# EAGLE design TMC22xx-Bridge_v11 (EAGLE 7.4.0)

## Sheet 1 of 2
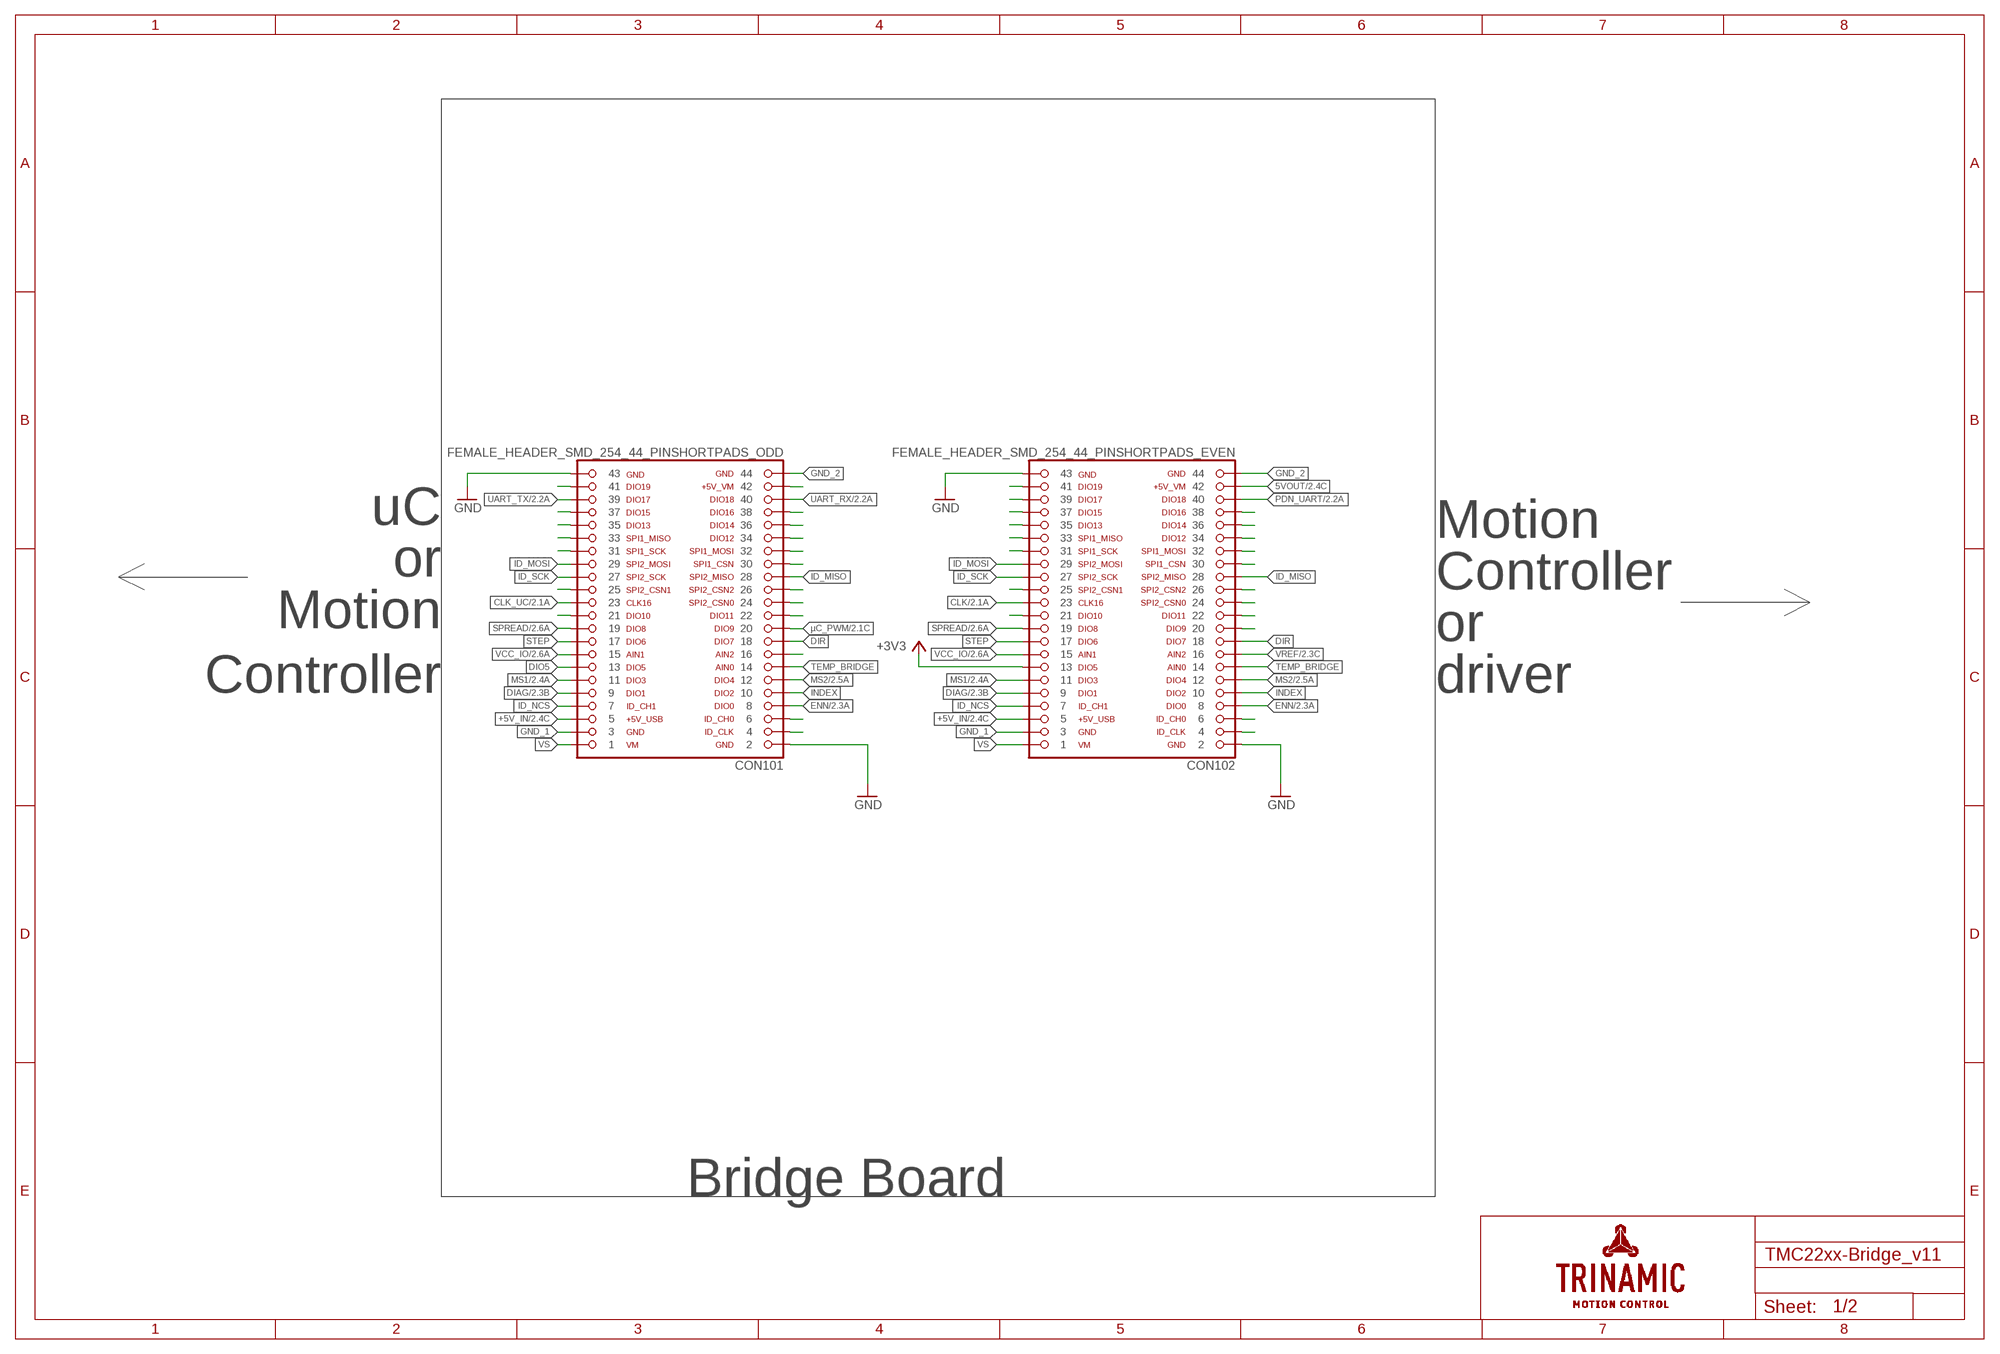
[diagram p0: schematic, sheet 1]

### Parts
CON101  FEMALE_HEADER_SMD_254_44_PINSHORTPADS_ODD  FEMALE_HEADER_SMD_2.54_44_PIN_BRIDGEESELSBRUECKE_ODD  [MALE_HEADER_SMD_254_44_PIN_SHORTPADS_ODD]
CON102  FEMALE_HEADER_SMD_254_44_PINSHORTPADS_EVEN  FEMALE_HEADER_SMD_2.54_44_PIN_BRIDGEESELSBRUECKE_EVEN  [MALE_HEADER_SMD_254_44_PIN_SHORTPADS_EVEN]

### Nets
5VOUT: CON102.1@42 CON102.42 ; also sheet 2
+3V3: CON102.13 ; also sheet 2
+5V_IN: CON101.1@5 CON101.5 CON102.5 ; also sheet 2
CLK: CON102.23 ; also sheet 2
CLK_UC: CON101.1@23 CON101.23 ; also sheet 2
DIAG: CON101.1@9 CON101.9 CON102.9 ; also sheet 2
DIO5: CON101.1@13 CON101.13
DIR: CON101.18 CON102.1@18 CON102.18
ENN: CON101.8 CON102.1@8 CON102.8 ; also sheet 2
GND: CON101.1@43 CON101.2 CON101.43 CON102.1@2 CON102.2 CON102.43 ; also sheet 2
GND_1: CON101.1@3 CON101.3 CON102.3
GND_2: CON101.44 CON102.1@44 CON102.44
ID_MISO: CON101.28 CON102.1@28 CON102.28
ID_MOSI: CON101.1@29 CON101.29 CON102.29
ID_NCS: CON101.1@7 CON101.7 CON102.7
ID_SCK: CON101.1@27 CON101.27 CON102.27
INDEX: CON101.10 CON102.1@10 CON102.10
MS1: CON101.1@11 CON101.11 CON102.11 ; also sheet 2
MS2: CON101.12 CON102.1@12 CON102.12 ; also sheet 2
N$4: CON101.1@41 CON101.41
N$6: CON101.1@37 CON101.37
N$7: CON101.1@35 CON101.35
N$8: CON101.1@33 CON101.33
N$9: CON101.1@31 CON101.31
N$10: CON101.1@25 CON101.25
N$11: CON101.1@21 CON101.21
N$13: CON101.4
N$14: CON101.6
N$15: CON101.22
N$16: CON101.26
N$17: CON101.24
N$18: CON101.30
N$19: CON101.32
N$20: CON101.34
N$21: CON101.36
N$22: CON101.38
N$23: CON101.42
N$24: CON102.41
N$25: CON102.39
N$26: CON102.37
N$27: CON102.35
N$28: CON102.33
N$29: CON102.31
N$30: CON102.25
N$31: CON102.21
N$33: CON102.1@4 CON102.4
N$34: CON102.1@6 CON102.6
N$35: CON102.1@20 CON102.20
N$36: CON102.1@22 CON102.22
N$37: CON102.1@24 CON102.24
N$38: CON102.1@26 CON102.26
N$39: CON102.1@30 CON102.30
N$40: CON102.1@32 CON102.32
N$41: CON102.1@34 CON102.34
N$42: CON102.1@36 CON102.36
N$43: CON102.1@38 CON102.38
PDN_UART: CON102.1@40 CON102.40 ; also sheet 2
SPREAD: CON101.1@19 CON101.19 CON102.19 ; also sheet 2
STEP: CON101.1@17 CON101.17 CON102.17
TEMP_BRIDGE: CON101.14 CON102.1@14 CON102.14
UART_RX: CON101.40 ; also sheet 2
UART_TX: CON101.1@39 CON101.39 ; also sheet 2
VCC_IO: CON101.1@15 CON101.15 CON102.15 ; also sheet 2
VREF: CON102.1@16 CON102.16 ; also sheet 2
VREF_NC: CON101.16
VS: CON101.1 CON101.1@1 CON102.1
µC_PWM: CON101.20 ; also sheet 2

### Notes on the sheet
- uC
- or | Motion
- Motion | Controller
- Controller | or
- driver
- Bridge Board

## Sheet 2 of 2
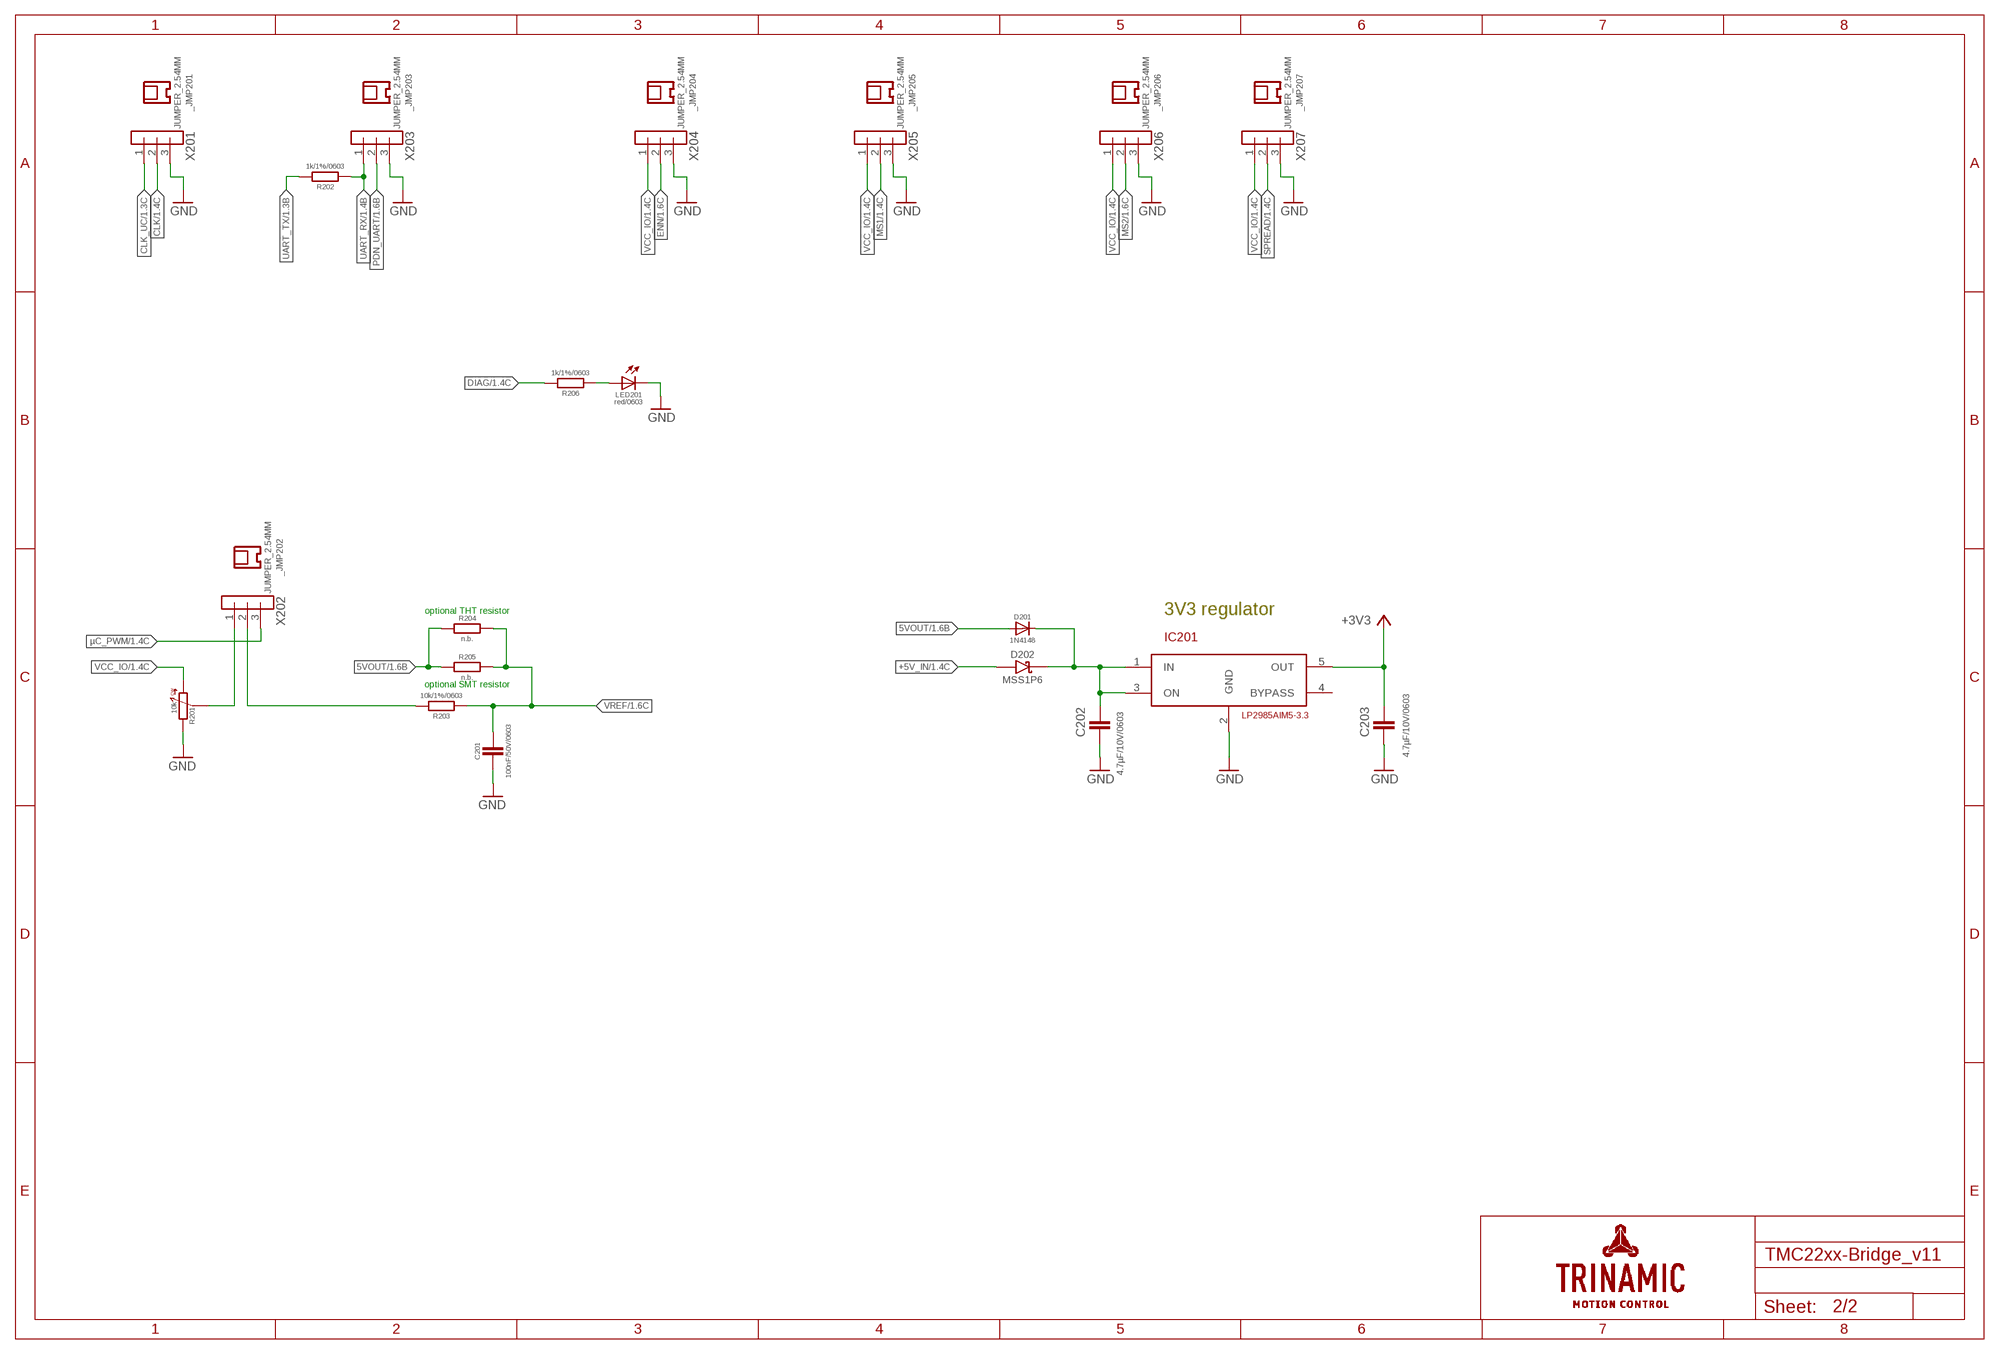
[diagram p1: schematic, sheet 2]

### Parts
_JMP201  JUMPER_2.54MM  [JUMPER_DOKU]
_JMP202  JUMPER_2.54MM  [JUMPER_DOKU]
_JMP203  JUMPER_2.54MM  [JUMPER_DOKU]
_JMP204  JUMPER_2.54MM  [JUMPER_DOKU]
_JMP205  JUMPER_2.54MM  [JUMPER_DOKU]
_JMP206  JUMPER_2.54MM  [JUMPER_DOKU]
_JMP207  JUMPER_2.54MM  [JUMPER_DOKU]
C201  100nF/50V/0603  C0603  [_RC_0603]
C202  4.7µF/10V/0603  C0603  [_RC_0603]
C203  4.7µF/10V/0603  C0603  [_RC_0603]
D201  1N4148  [D0603]
D202  MSS1P6  [MICROSMP]
IC201  LP2985AIM5-3.3  [SOT23-5]
LED201  red/0603  LED0603  [_D_0603]
R201  10k  CT-6EP  [COPAL-CT-6]
R202  1k/1%/0603  R0603  [_RC_0603]
R203  10k/1%/0603  R0603  [_RC_0603]
R204  n.b.  R-EU_0613/5V  [P0613V]
R205  n.b.  R_NOCREAM  [_RC_1206_NOCREAM]
R206  1k/1%/0603  R0603  [_RC_0603]
X201  3PIN_1ROWTHT  [3PIN_1ROM_2,54_THT]
X202  3PIN_1ROWTHT  [3PIN_1ROM_2,54_THT]
X203  3PIN_1ROWTHT  [3PIN_1ROM_2,54_THT]
X204  3PIN_1ROWTHT  [3PIN_1ROM_2,54_THT]
X205  3PIN_1ROWTHT  [3PIN_1ROM_2,54_THT]
X206  3PIN_1ROWTHT  [3PIN_1ROM_2,54_THT]
X207  3PIN_1ROWTHT  [3PIN_1ROM_2,54_THT]

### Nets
5V_TO_REG: C202.P$1 D201.K(C) D202.C IC201.1(IN) IC201.3(ON)
5VOUT: D201.A R204.1 R205.P$1 ; also sheet 1
+3V3: C203.P$1 IC201.5(OUT) ; also sheet 1
+5V_IN: D202.A ; also sheet 1
CLK: X201.2 ; also sheet 1
CLK_UC: X201.1 ; also sheet 1
DIAG: R206.P$2 ; also sheet 1
ENN: X204.2 ; also sheet 1
GND: C201.P$2 C202.P$2 C203.P$2 IC201.2(GND) LED201.C R201.P$1 X201.3 X203.3 X204.3 X205.3 X206.3 X207.3 ; also sheet 1
MS1: X205.2 ; also sheet 1
MS2: X206.2 ; also sheet 1
N$5: LED201.A R206.P$1
PDN_UART: X203.2 ; also sheet 1
SPREAD: X207.2 ; also sheet 1
UART_RX: R202.P$1 X203.1 ; also sheet 1
UART_TX: R202.P$2 ; also sheet 1
VCC_IO: R201.P$3 X204.1 X205.1 X206.1 X207.1 ; also sheet 1
VREF: C201.P$1 R203.P$1 R204.2 R205.P$2 ; also sheet 1
VREF_POT: R201.P$2 X202.1
VREF_POT_JP: R203.P$2 X202.2
µC_PWM: X202.3 ; also sheet 1
Unconnected: IC201.4(BYPASS)

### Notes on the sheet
- optional THT resistor | 3V3 regulator
- optional SMT resistor

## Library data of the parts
_JMP201-_JMP207 = TMC2208-Eval:JUMPER_2.54MM: Jumper 2.54mm, Open top, h6.5mm, black
C201-C203 = TMC2208-Eval:C
CON101 CON102 = TMC2208-Eval:FEMALE_HEADER_SMD_2.54_44_PIN_BRIDGE; SUPPLIER: MPE Garry; SUPPLIER-CODE: 090-3-044-1-F-XT0-0910
D201 = TMC2208-Eval:1N4148: DIODE; OC_DIGIKEY: 641-1001-1-ND; SUPPLIER: DigiKey; SUPPLIER-CODE: 641-1001-1-ND
D202 = TMC2208-Eval:MSS1P6; OC_DIGIKEY: MSS1P6-M3/89AGICT-ND; SUPPLIER: DigiKey; SUPPLIER-CODE: MSS1P6-M3/89AGICT-ND
IC201 = TMC2208-Eval:LP2985AIM5-3.3; OC_DIGIKEY: LP2985AIM5-3.3/NOPBCT-ND; SUPPLIER: DigiKey; SUPPLIER-CODE: LP2985AIM5-3.3/NOPBCT-ND
LED201 = TMC2208-Eval:LED
R201 = TMC2208-Eval:CT-6EP: Copal CT-6EP Potentiometer; OC_DIGIKEY: CT6EP103-ND; SUPPLIER: DigiKey; SUPPLIER-CODE: CT6EP103-ND
R202 R203 R206 = TMC2208-Eval:R
R204 = TMC2208-Eval:R-EU_: RESISTOR, European symbol
R205 = TMC2208-Eval:R_NOCREAM
X201-X207 = TMC2208-Eval:3PIN_1ROW

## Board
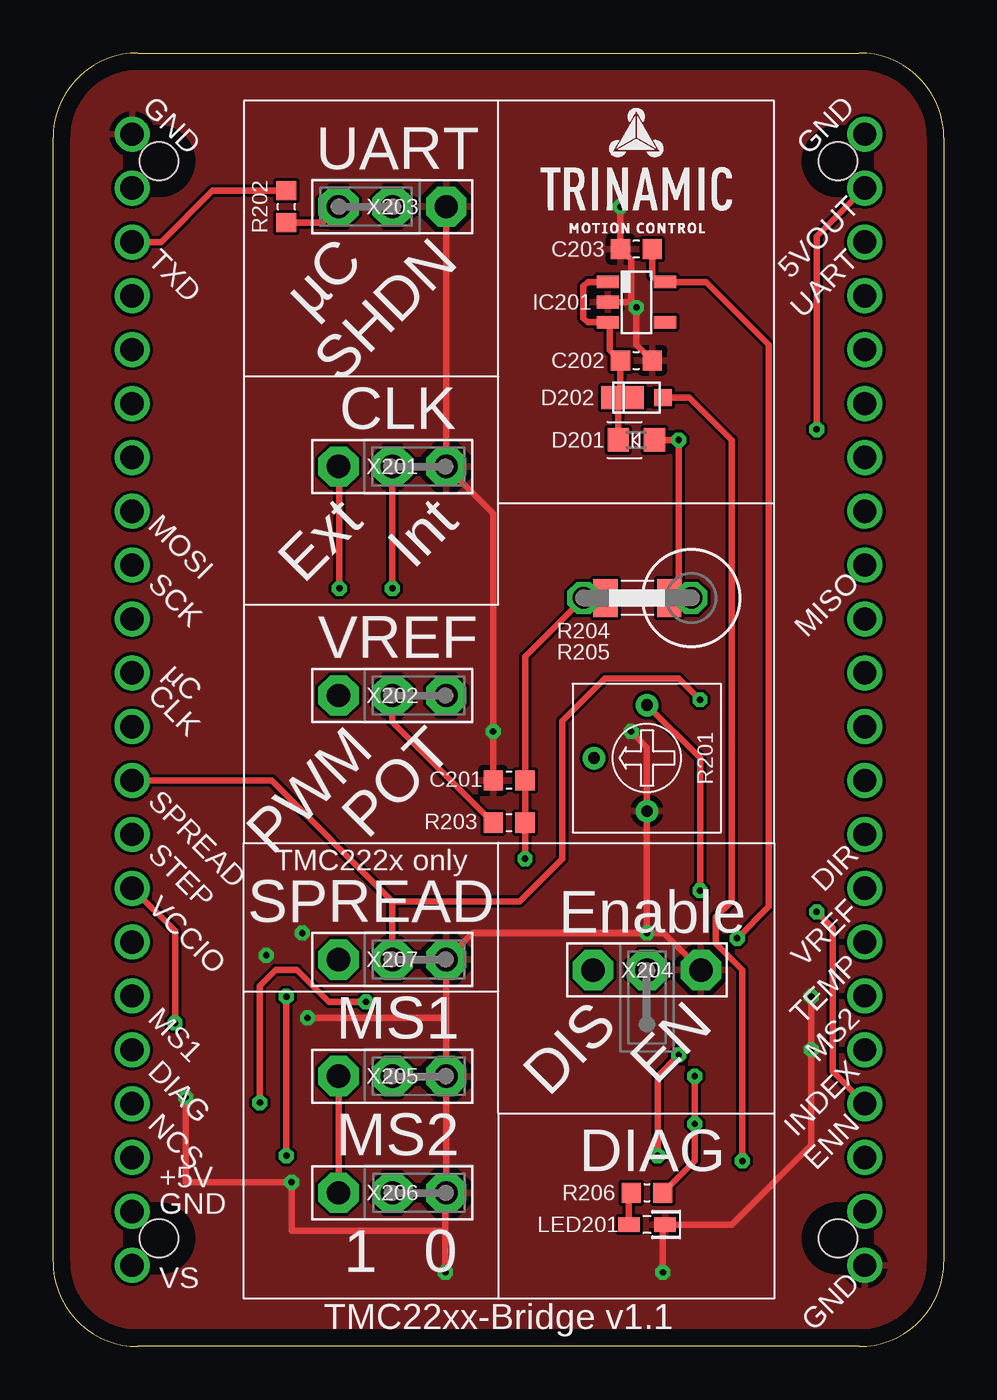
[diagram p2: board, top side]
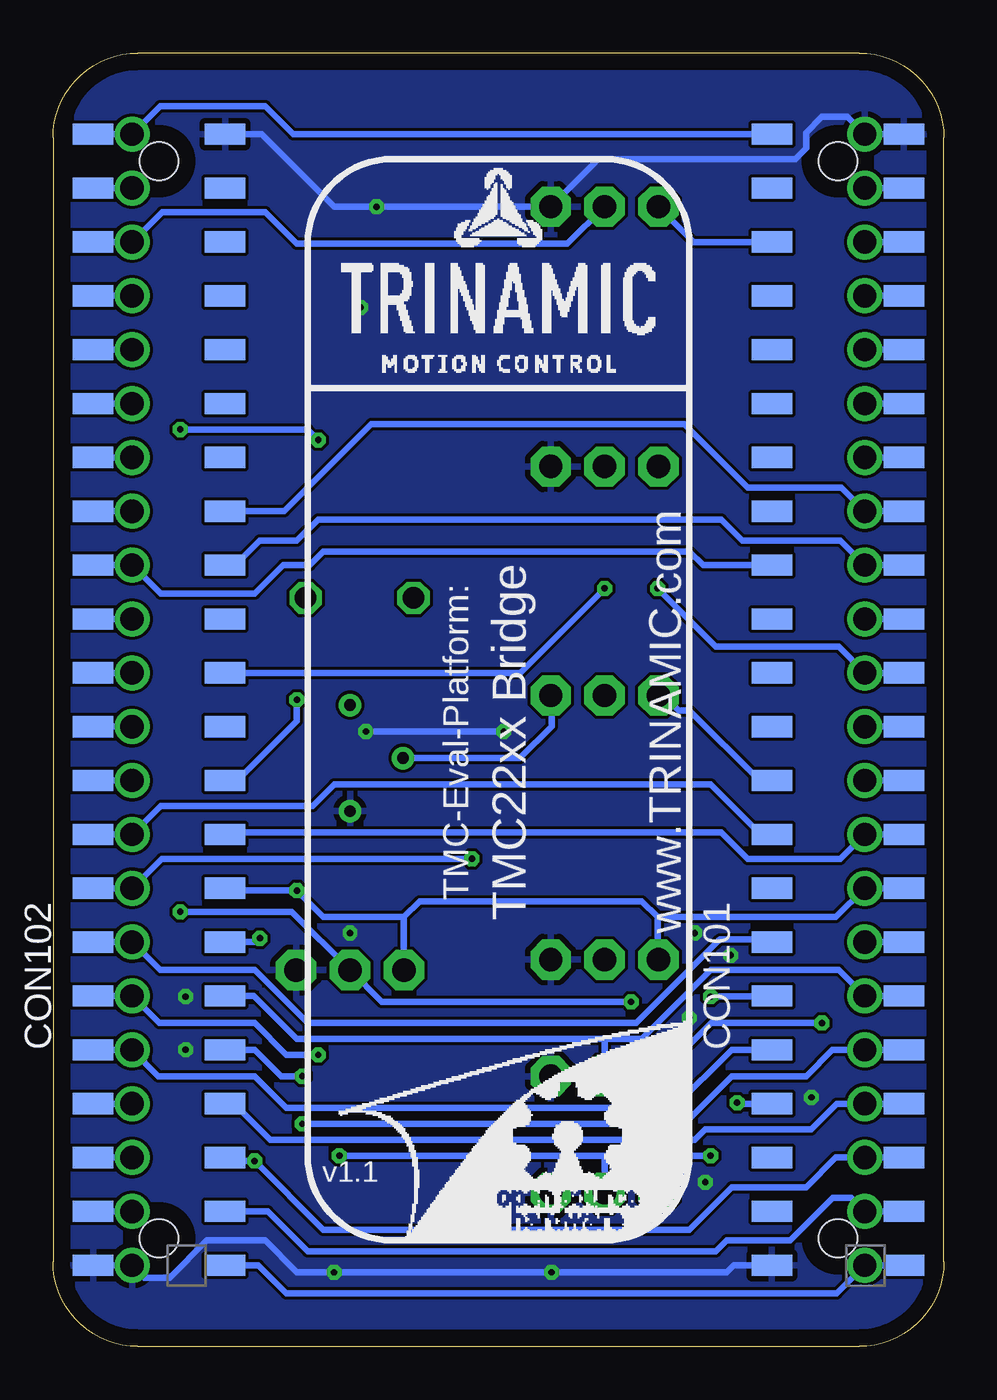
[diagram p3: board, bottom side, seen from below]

Size 42 x 61 mm. Coordinates in mm from the lower left corner, seen from the top.
Outline: 38,0 4,0 arc-90 0,4 0,57 arc-90 4,61 38,61 arc-90 42,57 42,4 arc-90 38,0
Copper layers (1*16): Top 0.018mm / dielectric 0.36mm / Bottom 0.018mm
Design rules "default": minimum track width 0.15mm, minimum drill 0.25mm, track to track 0.15mm, track to pad 0.15mm, pad to pad 0.1mm, via to via 0.15mm, smd to smd 0mil, copper to edge 0.8mm, drill to drill 8mil, minimum pad ring 10mil, minimum via ring 8mil, stop-mask expansion 4mil, vias tented up to drill 0.4mm, thermal gap 10mil

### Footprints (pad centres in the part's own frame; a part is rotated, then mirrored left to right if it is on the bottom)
_RC_0603 = smd 0.9 x 0.95: P$1 -0.75,0; P$2 0.75,0
MALE_HEADER_SMD_254_44_PIN_SHORTPADS_ODD = smd 1 x 1.9: 1 -26.67,-3.11; 2 -26.67,3.11; 3 -24.13,-3.11; 4 -24.13,3.11; 5 -21.59,-3.11; 6 -21.59,3.11; 7 -19.05,-3.11; 8 -19.05,3.11; 9 -16.51,-3.11; 10 -16.51,3.11; 11 -13.97,-3.11; 12 -13.97,3.11; 13 -11.43,-3.11; 14 -11.43,3.11; 15 -8.89,-3.11; 16 -8.89,3.11; 17 -6.35,-3.11; 18 -6.35,3.11; 19 -3.81,-3.11; 20 -3.81,3.11; 21 -1.27,-3.11; 22 -1.27,3.11; 23 1.27,-3.11; 24 1.27,3.11; 25 3.81,-3.11; 26 3.81,3.11; 27 6.35,-3.11; 28 6.35,3.11; 29 8.89,-3.11; 30 8.89,3.11; 31 11.43,-3.11; 32 11.43,3.11; 33 13.97,-3.11; 34 13.97,3.11; 35 16.51,-3.11; 36 16.51,3.11; 37 19.05,-3.11; 38 19.05,3.11; 39 21.59,-3.11; 40 21.59,3.11; 41 24.13,-3.11; 42 24.13,3.11; 43 26.67,-3.11; 44 26.67,3.11 | drill 1.1 pad 1.45: 1@1 -26.67,-1.27; 1@3 -24.13,-1.27; 1@5 -21.59,-1.27; 1@7 -19.05,-1.27; 1@9 -16.51,-1.27; 1@11 -13.97,-1.27; 1@13 -11.43,-1.27; 1@15 -8.89,-1.27; 1@17 -6.35,-1.27; 1@19 -3.81,-1.27; 1@21 -1.27,-1.27; 1@23 1.27,-1.27; 1@25 3.81,-1.27; 1@27 6.35,-1.27; 1@29 8.89,-1.27; 1@31 11.43,-1.27; 1@33 13.97,-1.27; 1@35 16.51,-1.27; 1@37 19.05,-1.27; 1@39 21.59,-1.27; 1@41 24.13,-1.27; 1@43 26.67,-1.27 | hole 1.8: -25.4,0; 25.4,0
MALE_HEADER_SMD_254_44_PIN_SHORTPADS_EVEN = smd 1 x 1.9: 1 -26.67,-3.11; 2 -26.67,3.11; 3 -24.13,-3.11; 4 -24.13,3.11; 5 -21.59,-3.11; 6 -21.59,3.11; 7 -19.05,-3.11; 8 -19.05,3.11; 9 -16.51,-3.11; 10 -16.51,3.11; 11 -13.97,-3.11; 12 -13.97,3.11; 13 -11.43,-3.11; 14 -11.43,3.11; 15 -8.89,-3.11; 16 -8.89,3.11; 17 -6.35,-3.11; 18 -6.35,3.11; 19 -3.81,-3.11; 20 -3.81,3.11; 21 -1.27,-3.11; 22 -1.27,3.11; 23 1.27,-3.11; 24 1.27,3.11; 25 3.81,-3.11; 26 3.81,3.11; 27 6.35,-3.11; 28 6.35,3.11; 29 8.89,-3.11; 30 8.89,3.11; 31 11.43,-3.11; 32 11.43,3.11; 33 13.97,-3.11; 34 13.97,3.11; 35 16.51,-3.11; 36 16.51,3.11; 37 19.05,-3.11; 38 19.05,3.11; 39 21.59,-3.11; 40 21.59,3.11; 41 24.13,-3.11; 42 24.13,3.11; 43 26.67,-3.11; 44 26.67,3.11 | drill 1.1 pad 1.45: 1@2 -26.67,1.27; 1@4 -24.13,1.27; 1@6 -21.59,1.27; 1@8 -19.05,1.27; 1@10 -16.51,1.27; 1@12 -13.97,1.27; 1@14 -11.43,1.27; 1@16 -8.89,1.27; 1@18 -6.35,1.27; 1@20 -3.81,1.27; 1@22 -1.27,1.27; 1@24 1.27,1.27; 1@26 3.81,1.27; 1@28 6.35,1.27; 1@30 8.89,1.27; 1@32 11.43,1.27; 1@34 13.97,1.27; 1@36 16.51,1.27; 1@38 19.05,1.27; 1@40 21.59,1.27; 1@42 24.13,1.27; 1@44 26.67,1.27 | hole 1.8: -25.4,0; 25.4,0
D0603 = smd 1 x 1.1: A -0.85,0; K 0.85,0
MICROSMP = smd 0.813 x 0.813: A 1.257,0 | smd 2.007 x 1.092: C -0.66,0
SOT23-5 = smd 0.6 x 1.05: 1 -0.95,-1.35; 2 0,-1.35; 3 0.95,-1.35; 4 0.95,1.35; 5 -0.95,1.35
_D_0603 = smd 1 x 0.7: A 0.85,0; C -0.85,0
COPAL-CT-6 = drill 0.55: P$1 -2.5,0; P$2 0,2.5; P$3 2.5,0
P0613V = drill 1.016 octagon: 1 -2.54,0; 2 2.54,0
_RC_1206_NOCREAM = smd 1.15 x 1.8: P$1 -1.5,0; P$2 1.5,0
3PIN_1ROM_2,54_THT = drill 1.1 pad 1.9 octagon: 1 -2.54,0; 2 0,0; 3 2.54,0

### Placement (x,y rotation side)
_JMP201  17.23,18.25 0 top
_JMP202  28,16.46 90 top
_JMP203  17.24,12.75 0 top
_JMP204  17.25,7.25 0 top
_JMP205  17.23,30.7 0 top
_JMP206  17.22,41.5 0 top
_JMP207  14.75,53.75 0 top
C201  21.5,26.7 180 top
C202  27.5,46.5 0 top
C203  27.5,51.75 180 top
CON101  5,30.5 90 bottom
CON102  37,30.5 90 bottom
D201  27.5,42.75 180 top
D202  27.5,44.75 0 top
IC201  27.5,49.25 270 top
LED201  28,5.75 180 top
R201  28,27.75 90 top
R202  11,53.75 90 top
R203  21.5,24.7 180 top
R204  27.55,35.3 180 top
R205  27.55,35.3 180 top
R206  28,7.25 0 top
U$3  [TRINAMIC_LOGO]  23,52.5 0 top
U$4  [TMC_EVAL_BACK_BRIDGE]  30,5 0 bottom
X201  16,41.5 0 top
X202  16,30.7 180 top
X203  16,53.75 0 top
X204  28,17.75 0 top
X205  16,12.75 0 top
X206  16,7.25 0 top
X207  16,18.25 0 top

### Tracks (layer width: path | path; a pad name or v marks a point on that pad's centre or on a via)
5V_TO_REG
  Top 0.3: IC201.1 25.2,50.2 25,50 25,48.5 25.2,48.3 IC201.3 26.25,48.2 26.25,47 C202.P$1 26.75,44.84 D202.C 26.65,44.56 D201.K
5VOUT  (via drill 0.3)
  Top 0.3: R204.1 R205.P$1 29.5,35.75 v29.5,42.75 D201.A | CON102.1@42 36,52.36 v36,43.25
  Bottom 0.3: CON102.42 CON102.1@42 | v36,43.25 30,43.25 v29.5,42.75
+3V3  (via drill 0.3)
  Top 0.3: C203.P$1 28.25,50.5 28.55,50.2 IC201.5 30.8,50.2 33.75,47.25 33.75,20.75 v32.25,19.25
  Bottom 0.3: CON102.13 32.43,19.07 v32.25,19.25
+5V_IN  (via drill 0.3)
  Top 0.3: v32.5,8.75 32.5,17.75 31.25,19 31.25,20.25 32,21 32,42.75 30,44.75 D202.A
  Bottom 0.3: CON101.5 CON101.1@5 5.09,8.91 6.5,7.5 10,7.5 12,5.5 29.25,5.5 v32.5,8.75 33.73,8.75 CON102.5
CLK  (via drill 0.3)
  Top 0.3: v16,35.75 X201.2
  Bottom 0.3: 33.87,31.75 CON102.23 19.98,31.77 v16,35.75
CLK_UC  (via drill 0.3)
  Top 0.3: X201.1 13.5,41.46 v13.5,35.75
  Bottom 0.3: CON101.23 CON101.1@23 4.96,33 10.75,33 v13.5,35.75
DIAG  (via drill 0.3)
  Top 0.3: R206.P$2 30.25,8.75 v30.25,10.5 v30.25,12.75
  Bottom 0.3: CON101.9 CON101.1@9 5.26,13.99 6.5,12.75 10,12.75 12.25,10.5 v30.25,10.5 | CON102.9 32.49,13.99 31.25,12.75 v30.25,12.75
DIO5
  Bottom 0.3: CON101.13 CON101.1@13
DIR
  Bottom 0.3: CON102.18 CON102.1@18 36.92,25.5 29.75,25.5 28.75,26.5 11,26.5 8.5,24 8.26,24 CON101.18
ENN  (via drill 0.3)
  Top 0.3: v36,20.5 36.75,19.75 36.75,12.97 CON102.1@8 | v14.75,16.25 13,16.25 11.5,17.75 10.5,17.75 9.75,17 v9.75,11.5
  Bottom 0.3: CON102.8 CON102.1@8 | v36,20.5 30.75,20.5 X204.2 26.5,16.25 v14.75,16.25 | v9.75,11.5 9.7,11.45 CON101.8
GND  (via drill 0.3)
  Top 0.3: 27.25,49.25 27.25,51.25 C203.P$2 v26.75,53.75 | 27.25,49.25 IC201.2 | C202.P$2 27.5,47.25 v27.5,49 27.25,49.25 | C201.P$2 v20.75,29 20.75,39.29 X201.3 X203.3 | v27.25,29 28,28.25 R201.P$1 v28,19.5 | v28.75,3.5 28.75,5.65 LED201.C 32,5.75 35.75,9.5 v35.75,14 v35.75,16.5 | 18.5,5.45 18.5,7.21 X206.3 X205.3 18.54,15.5 | 18.5,5.45 v18.5,3.5 | v28,19.5 19.79,19.5 X207.3 18.54,15.5 | X204.3 28.79,19.5 v28,19.5 | 18.54,15.5 v12,15.5 | 18.5,5.45 11.25,5.45 v11.25,7.75 6.25,7.75 v6.25,11.75
  Bottom 0.3: CON101.43 CON101.1@43 4.56,58 5.75,58 6.5,57.25 6.5,56.5 7,56 16.29,56 X203.3 v26.75,53.75 28.75,53.75 32.17,57.17 CON102.43 | v27.25,29 v20.75,29 | CON102.2 CON102.1@2 37.69,3.25 36.5,3.25 34.75,5 32,5 30.5,3.5 v28.75,3.5 v18.5,3.5 10.25,3.5 9.92,3.83 CON101.2
  other vias: 11.75,19.5 10.05,18.45
  pour Bottom: 42,61 0,61 0,0 42,0
  pour Top: 42,61 0,61 0,0 42,0
GND_1
  Bottom 0.3: CON101.3 CON101.1@3 4.36,7 5.25,7 7.25,5 10.25,5 10.75,4.5 30,4.5 31.87,6.37 CON102.3
GND_2
  Bottom 0.3: CON102.44 CON102.1@44 36.94,58.5 32,58.5 30.67,57.17 CON101.44
ID_MISO
  Bottom 0.3: CON102.28 CON102.1@28 36.92,35.5 32.5,35.5 31.15,36.85 29.9,36.85 29.25,37.5 12,37.5 11.35,36.85 CON101.28
ID_MOSI
  Bottom 0.3: CON101.29 CON101.1@29 4.84,40.5 9.25,40.5 12.25,43.5 27,43.5 31.11,39.39 CON102.29
ID_NCS
  Bottom 0.3: CON101.7 CON101.1@7 5.05,11.45 6.25,10.25 11.25,10.25 11.75,9.75 31.75,9.75 33.45,11.45 CON102.7
ID_SCK
  Bottom 0.3: CON101.27 CON101.1@27 4.88,38 9.5,38 10.5,39 29.5,39 30.5,38 32.25,38 33.4,36.85 CON102.27
INDEX
  Bottom 0.3: CON102.10 CON102.1@10 37.03,12.75 32.5,12.75 31,11.25 12.75,11.25 10.01,13.99 CON101.10
MS1
  Bottom 0.3: CON101.11 CON101.1@11 4.95,17.75 11,17.75 14.25,14.5 16,14.5 | CON102.11 32.53,16.53 30.5,14.5 16,14.5 | X205.2 16,14.5
MS2  (via drill 0.3)
  Top 0.3: v28.5,9 28.5,12.75 v29.5,13.75 | v11,9 v11,16.5
  Bottom 0.3: CON102.12 CON102.1@12 36.99,15.25 32.5,15.25 31,13.75 v29.5,13.75 | 16,9 v28.5,9 | 16,9 X206.2 | 16,9 v11,9 | v11,16.5 8.14,16.5 CON101.12
N$4
  Bottom 0.3: CON101.41 CON101.1@41
N$5
  Top 0.3: LED201.A 27.15,7.15 R206.P$1
N$6
  Bottom 0.3: CON101.37 CON101.1@37
N$7
  Bottom 0.3: CON101.35 CON101.1@35
N$8
  Bottom 0.3: CON101.33 CON101.1@33
N$9
  Bottom 0.3: CON101.31 CON101.1@31
N$10
  Bottom 0.3: CON101.25 CON101.1@25
N$11
  Bottom 0.3: CON101.21 CON101.1@21
N$33
  Bottom 0.3: CON102.4 CON102.1@4
N$34
  Bottom 0.3: CON102.6 CON102.1@6
N$35
  Bottom 0.3: CON102.20 CON102.1@20
N$36
  Bottom 0.3: CON102.22 CON102.1@22
N$37
  Bottom 0.3: CON102.24 CON102.1@24
N$38
  Bottom 0.3: CON102.26 CON102.1@26
N$39
  Bottom 0.3: CON102.30 CON102.1@30
N$40
  Bottom 0.3: CON102.32 CON102.1@32
N$41
  Bottom 0.3: CON102.34 CON102.1@34
N$42
  Bottom 0.3: CON102.36 CON102.1@36
N$43
  Bottom 0.3: CON102.38 CON102.1@38
PDN_UART
  Bottom 0.3: CON102.40 CON102.1@40 36.86,53.5 32,53.5 30.5,52 17.75,52 X203.2
SPREAD  (via drill 0.3)
  Top 0.3: v30.5,30.5 29.5,31.5 26,31.5 24,29.5 24,23 22,21 16,21 | 16,21 X207.2 | CON101.1@19 10.31,26.69 16,21
  Bottom 0.3: CON101.19 CON101.1@19 | CON102.19 33.31,26.69 30.5,29.5 v30.5,30.5
STEP
  Bottom 0.3: CON101.17 CON101.1@17 4.88,23 9.25,23 10.5,24.25 33.79,24.25 CON102.17
TEMP_BRIDGE
  Bottom 0.3: CON102.14 CON102.1@14 36.95,17.75 32.5,17.75 30,15.25 14.5,15.25 10.75,19 10.63,19.12 10.55,19.2 8.24,19.2 CON101.14
UART_RX
  Top 0.3: R202.P$1 12.71,53 X203.1
  Bottom 0.3: CON101.40 11.8,52.09 X203.1
UART_TX
  Top 0.3: R202.P$2 7.5,54.5 5.09,52.09 CON101.1@39
  Bottom 0.3: CON101.39 CON101.1@39
VCC_IO  (via drill 0.3)
  Top 0.3: X206.1 X205.1 | v5.75,15.25 5.75,19.59 CON101.1@15 | v30.5,21.5 30.5,27.75 R201.P$3
  Bottom 0.3: CON101.15 CON101.1@15 5.09,20.25 13.5,20.25 | X205.1 10.96,15.25 v5.75,15.25 | 25.46,20.25 X204.1 | 25.46,20.25 29.25,20.25 v30.5,21.5 33.78,21.5 CON102.15 | X207.1 13.5,18.29 13.5,20.25 | 13.5,20.25 14.25,21 24.71,21 25.46,20.25
VREF  (via drill 0.3)
  Top 0.3: R205.P$2 R204.2 22.25,32.54 C201.P$1 R203.P$1 v22.25,23
  Bottom 0.3: CON102.16 CON102.1@16 36.88,23 v22.25,23
VREF_POT
  Bottom 0.3: R201.P$2 20,27.75 18.5,29.25 18.5,30.66 X202.1
VREF_POT_JP
  Top 0.3: R203.P$2 16,29.45 X202.2
VS
  Bottom 0.3: CON101.1 CON101.1@1 5.06,2.5 31,2.5 32.33,3.83 CON102.1
µC_PWM
  Bottom 0.3: CON101.20 8.69,26.69 12,30 12.5,30 13.2,30.7 X202.3

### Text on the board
tPlace: GND | GND | UART | 5VOUT | TXD | µC | SHDN | UART | CLK | Ext | Int | MOSI | SCK | MISO | µC | VREF | CLK | PWM | POT | SPREAD | STEP | DIR | TMC222x only | VCCIO | VREF | SPREAD | Enable | TEMP | MS1 | DIS | EN | MS2 | MS1 | DIAG | INDEX | NCS | ENN | MS2 | +5V | DIAG | GND | 1 | 0 | VS | GND | TMC22xx-Bridge v1.1
bPlace: TMC22xx Bridge | TMC-Eval-Platform: | v1.1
